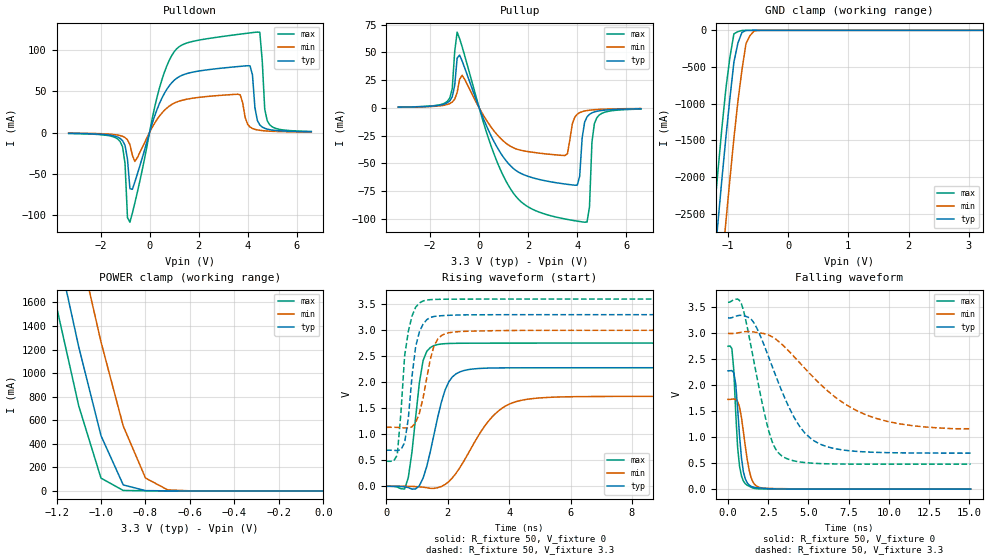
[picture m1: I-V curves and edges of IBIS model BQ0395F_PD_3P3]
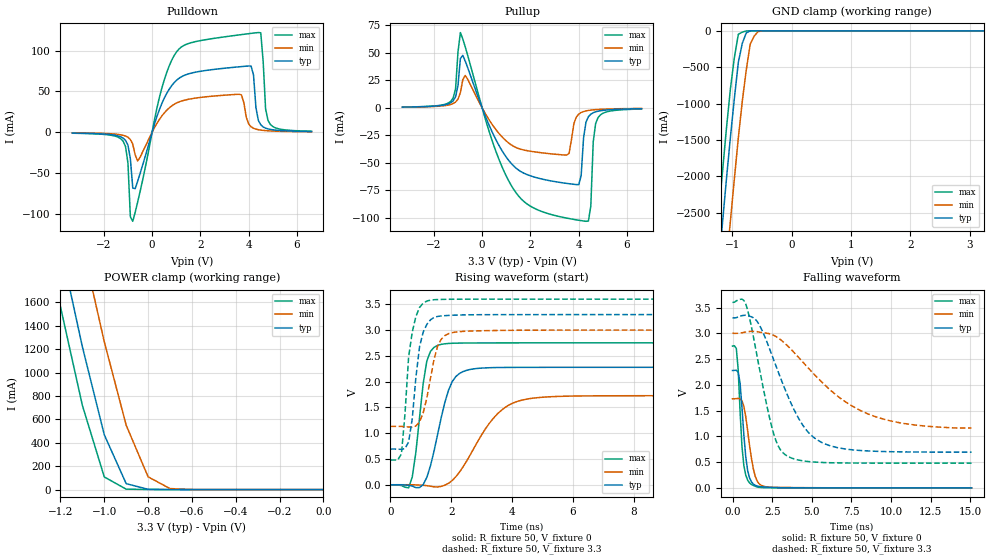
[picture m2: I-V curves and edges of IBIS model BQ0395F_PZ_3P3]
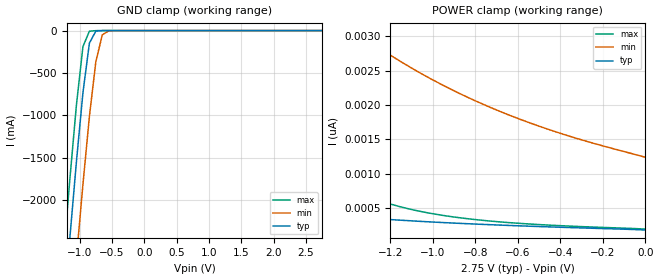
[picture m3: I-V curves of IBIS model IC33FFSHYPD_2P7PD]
[IBIS Ver]   3.2
[File Name]   sprm398.ibs
[File Rev]   1.0
[Date]   February 11, 2008
[Source]   File originated at Texas Instruments
[Copyright]   (c) 2008, Texas Instruments Inc.
[Component]   f2802xpt
[Manufacturer] Texas Instruments
[Package]
| Variable   Typ   Min   Max
R_pkg   0.277   0.133   0.378
L_pkg   1.76e-09   1.23e-09   2.19e-09
C_pkg   0.146e-12   0.05e-12   0.274e-12
[Pin] signal_name   model_name   R_pin   L_pin   C_pin
1   GPIO29   BQ0395F   0.284  1.74e-09  0.121e-12
2   TRSTn   IC33FFSHYPD   0.254  1.59e-09  0.167e-12
3   XRSn   BC3350BFODHYPU   0.134  1.23e-09  0.172e-12
4   ADCINA6   NC   0.290  1.69e-09  0.156e-12
5   ADCINA4   NC   0.150  1.46e-09  0.167e-12
6   ADCINA7   NC   0.260  1.67e-09  0.094e-12
7   ADCINA3   NC   0.248  1.54e-09  0.139e-12
8   ADCINA1   NC   0.244  1.53e-09  0.145e-12
9   ADCINA2   NC   0.252  1.51e-09  0.153e-12
10   ADCINA0   NC   0.151  1.39e-09  0.183e-12
11   VDDA   NC   0.286  1.83e-09  0.167e-12
12   VSSA   NC   0.163  1.61e-09  0.138e-12
13   ADCINB1   NC   0.315  1.87e-09  0.121e-12
14   ADCINB2   NC   0.314  1.84e-09  0.170e-12
15   ADCINB3   NC   0.317  1.870e-09 0.163e-12
16   ADCINB4   NC   0.323  1.86e-09  0.155e-12
17   ADCINB6   NC   0.330  1.80e-09  0.149e-12
18   ADCINB7   NC   0.343  1.86e-09  0.057e-12
19   GPIO34   BC3350AFHYPU   0.336  1.87e-09  0.085e-12
20   GPIO35   BC3350AFHYPU   0.335  1.88e-09  0.147e-12
21   GPIO36   BC3325CFHYPU   0.336  1.98e-09  0.156e-12
22   GPIO37   BC3325CFHYPU   0.338  2.03e-09  0.164e-12
23   GPIO38   BC3350AFHYPU   0.337  1.94e-09  0.171e-12
24   GPIO18   BQ0395F   0.345  2.08e-09  0.123e-12
25   GPIO19   BC3325CFHYPU   0.291  1.82e-09  0.120e-12
26   GPIO17   BQ0395F   0.244  1.55e-09  0.167e-12
27   GPIO16   BQ0395F   0.238  1.48e-09  0.156e-12
28   GPIO1   BQ0483F   0.235  1.36e-09  0.149e-12
29   GPIO0   BQ0393F   0.242  1.51e-09  0.145e-12
30   TEST   NC   0.249  1.55e-09  0.089e-12
31   GPIO32   BQ0393F   0.247  1.55e-09  0.081e-12
32   VDD   NC   0.251  1.62e-09  0.145e-12
33   VSS   NC   0.264  1.57e-09  0.155e-12
34   VREGENZn   NC   0.297  1.80e-09  0.165e-12
35   VDDIO   NC   0.156  1.52e-09  0.184e-12
36   GPIO33   BQ0393F   0.285  1.72e-09  0.119e-12
37   GPIO2   BQ0393F   0.314  1.95e-09  0.124e-12
38   GPIO3   BQ0393F   0.314  1.96e-09  0.175e-12
39   GPIO4   BQ0393F   0.324  1.89e-09  0.167e-12
40   GPIO5   BQ0393F   0.348  2.1e-09   0.159e-12
41   GPIO6   BQ0393F   0.346  2.09e-09  0.147e-12
42   GPIO7   BQ0393F   0.344  2.08e-09  0.085e-12
43   VDD   NC   0.133  1.64e-09  0.205e-12
44   VSS   NC   0.133  1.65e-09  0.207e-12
45   X1   NC   0.350  2.06e-09  0.163e-12
46   X2   NC   0.378  2.19e-09  0.171e-12
47   GPIO12   BQ0393F   0.315  1.95e-09  0.169e-12
48   GPIO28   BQ0395F   0.315  2.02e-09  0.1219e-12
| End of package information
[Component]   BQ0395F
[Manufacturer]   Texas Instruments
[Package]
|  variable   typ   min   max
R_pkg   0   0   0
L_pkg   0   0   0
C_pkg   0   0   0
[Pin]   signal_name   model_name   R_pin   L_pin   C_pin
VSS   VSS   GND
VDDS   VDDS   POWER
PAD   PAD   BQ0395F
[Model Selector] BQ0395F
BQ0395F_PD_3P3  Cell operated at 3.3(nom)
|BQ0395F_PD_3P3; PULLDOWN_ON
BQ0395F_PZ_3P3  Cell operated at 3.3(nom)
[Component]   IC33FFSHYPD
[Manufacturer]   Texas Instruments.
[Package]
| variable   typ   min   max
R_pkg   0.000   0.000   0.000
L_pkg   0.000H   0.000H   0.000H
C_pkg   0.000F   0.000F   0.000F
[Pin]  signal_name   model_name   R_pin   L_pin   C_pin
PAD   PAD   IC33FFSHYPD_3P3PD
| Y   Y   dummy
VSS   VSS   GND
VDDS   VDDS   POWER
[Model Selector]  IC33FFSHYPD
IC33FFSHYPD_2P7PD   cell with PI=0 and VDDS as 2.75(typ)
IC33FFSHYPD_2P7PDZ   cell with PI=1 and VDDS as 2.75(typ)
IC33FFSHYPD_3P3PD   cell with PI=0 and VDDS as 3.3(typ)
IC33FFSHYPD_3P3PDZ   cell with PI=1 and VDDS as 3.3(typ)
|   Component IC33FFSHYPU
[Component]   BC3350BFODHYPU
[Manufacturer]   Texas Instruments.
[Package]
| variable   typ   min   max
R_pkg   0.000   0.000   0.000
L_pkg   0.000H   0.000H   0.000H
C_pkg   0.000F   0.000F   0.000F
[Pin]  signal_name   model_name   R_pin   L_pin   C_pin
PAD   PAD   BC3350BFODHYPU_3P3PU
| A   A   dummy
| GZ   GZ   dummy
| Y   Y   dummy
VSSS   VSSS   GND
VDDS   VDDS   POWER
[Model Selector]   BC3350BFODHYPU
BC3350BFODHYPU_2P5PU   cell   VDDS=2.75(TYP)
BC3350BFODHYPU_2P5PZ   cell   VDDS=2.75(TYP)
BC3350BFODHYPU_3P3PU   cell   VDDS=3.3(TYP)
BC3350BFODHYPU_3P3PZ   cell   VDDS=3.3(TYP)
|   Component IC33FFSHY
[Component]   BC3350AFHYPU
[Manufacturer]   Texas Instruments.
[Package]
| variable   typ   min   max
R_pkg   0.000   0.000   0.000
L_pkg   0.000H   0.000H   0.000H
C_pkg   0.000F   0.000F   0.000F
[Pin]  signal_name   model_name   R_pin   L_pin   C_pin
PAD   PAD   BC3350AFHYPU_3P3PU
| A   A   dummy
| GZ   GZ   dummy
| Y   Y   dummy
VSSS   VSSS   GND
VDDS   VDDS   POWER
[Model Selector]  BC3350AFHYPU
BC3350AFHYPU_2P5PU   cell   VDDS=2.5V(typ)  PI=0
BC3350AFHYPU_2P5PUZ  cell   VDDS=2.5V(typ)  PI=1
BC3350AFHYPU_3P3PU   cell   VDDS=3.3V(typ)  PI=0
BC3350AFHYPU_3P3PUZ  cell   VDDS=3.3V(typ)  PI=1
|   Component OC3325CF
[Component]   BC3325CFHYPU
[Manufacturer]   Texas Instruments.
[Package]
| variable   typ   min   max
R_pkg   0.000   0.000   0.000
L_pkg   0.000H   0.000H   0.000H
C_pkg   0.000F   0.000F   0.000F
[Pin]  signal_name   model_name   R_pin   L_pin   C_pin
PAD   PAD   BC3325CFHYPU_3P3PU
| A   A   dummy
| GZ   GZ   dummy
| Y   Y   dummy
VSSS   VSSS   GND
VDDS   VDDS   POWER
[Model Selector]   BC3325CFHYPU
BC3325CFHYPU_2P5PU   cell  VDDS=2.75(TYP)  PI=0
BC3325CFHYPU_2P5PUZ   cell  VDDS=2.75(TYP)  PI=1
BC3325CFHYPU_3P3PU   cell  VDDS=3.3(TYP)  PI=0
BC3325CFHYPU_3P3PUZ   cell  VDDS=3.3(TYP)  PI=1
|   Component BC3350AFHYPU
[Component]   BQ0483F
[Manufacturer]   Texas Instruments
[Package]
|  variable   typ   min   max
R_pkg   0   0   0
L_pkg   0   0   0
C_pkg   0   0   0
[Pin]   signal_name   model_name   R_pin   L_pin   C_pin
VSS   VSS   GND
VDDS   VDDS   POWER
PAD   PAD   BQ0483F
[Model Selector] BQ0483F
BQ0483F_PD_3P3  Cell operated at 3.3(nom)
|BQ0483F_PD_3P3; PULLDOWN_ON
BQ0483F_PZ_3P3  Cell operated at 3.3(nom)
[Component]   BQ0393F
[Manufacturer]   Texas Instruments
[Package]
|  variable   typ   min   max
R_pkg   0   0   0
L_pkg   0   0   0
C_pkg   0   0   0
[Pin]   signal_name   model_name   R_pin   L_pin   C_pin
VSS   VSS   GND
VDDS   VDDS   POWER
PAD   PAD   BQ0393F
[Model Selector] BQ0393F
BQ0393F_PD_3P3  Cell operated at 3.3(nom)
|BQ0393F_PD_3P3; PULLDOWN_ON
BQ0393F_PZ_3P3  Cell operated at 3.3(nom)
| Models and submodels in the file (22): BQ0395F_PD_3P3 (I/O), BQ0395F_PZ_3P3 (I/O), IC33FFSHYPD_2P7PD (Input), IC33FFSHYPD_2P7PDZ (Input), IC33FFSHYPD_3P3PD (Input), IC33FFSHYPD_3P3PDZ (Input), BC3350BFODHYPU_2P5PU (I/O_open_drain), BC3350BFODHYPU_2P5PZ (I/O_open_drain), BC3350BFODHYPU_3P3PU (I/O_open_drain), BC3350BFODHYPU_3P3PZ (I/O_open_drain), BC3350AFHYPU_2P5PU (I/O), BC3350AFHYPU_2P5PUZ (I/O), BC3350AFHYPU_3P3PU (I/O), BC3350AFHYPU_3P3PUZ (I/O), BC3325CFHYPU_2P5PU (I/O), BC3325CFHYPU_2P5PUZ (I/O), BC3325CFHYPU_3P3PU (I/O), BC3325CFHYPU_3P3PUZ (I/O), BQ0483F_PD_3P3 (I/O), BQ0483F_PZ_3P3 (I/O), BQ0393F_PD_3P3 (I/O), BQ0393F_PZ_3P3 (I/O)
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|BQ0395F_PZ_3P3; PULLDOWN_OFF
|   Model Cell BQ0395F_PD_3P3
|BQ0395F_PD_3P3
[Model]   BQ0395F_PD_3P3
Model_type   I/O
Polarity   Non-Inverting
Enable   Active-Low
Vinl =  1.15
Vinh =  1.65
Cref =  15.0001pF
Rref =  101.0000M
Vref =  0V
Vmeas =  1.65
C_comp   1.2p   1.2p   1.2p
[Model Spec]
Vinl   1.15   1.05   1.15
Vinh   1.65   1.65   1.65
[Temperature Range]   25   125   -40
[Voltage Range]   3.3   3   3.6
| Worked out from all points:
|   slope of the pulldown table from 0 to 0.495 V, typ, clamps not added: 12 ohm
|   slope of the pullup table from 0 to 0.495 V, typ, clamps not added: 19.4 ohm
|   GND clamp passes 1 mA (typ) near -0.66 V on its own axis
|   POWER clamp passes 1 mA (typ) near -0.72 V on its own axis
|   rising waveform, R_fixture 50, V_fixture 0: 20-80 % time 553ps typ, 1.15ns min, 327ps max; typ from 0.001 V to 2.28 V
|   rising waveform, R_fixture 50, V_fixture 3.3: 20-80 % time 302ps typ, 400ps min, 286ps max; typ from 0.695 V to 3.3 V
|   falling waveform, R_fixture 50, V_fixture 0: 20-80 % time 372ps typ, 499ps min, 308ps max; typ from 2.28 V to 0.001 V
|   falling waveform, R_fixture 50, V_fixture 3.3: 20-80 % time 2.21ns typ, 4.03ns min, 1.26ns max; typ from 3.3 V to 0.695 V
[POWER_clamp]
|   voltage   I(typ)   I(min)   I(max)
-3.3V     22.47A     23.26A     22.03A
-1.233V   2.386A     3.273A     1.866A
-1.2V     2.084A     2.97A      1.564A
-1.167V   1.796A     2.677A     1.283A
-1.133V   1.509A     2.384A     1.002A
-1.067V   970.3mA    1.815A     516.3mA
-1.033V   719.4mA    1.539A     312.3mA
-1V       468.5mA    1.264A     108.3mA
-900mV    50.9mA     550mA      3.945mA
-800mV    2.599mA    109.2mA    1.152mA
-700mV    531.1uA    8.818mA    336.1uA
0V        279.6pA    1.919nA    325pA
[Pulldown]
|   voltage   I(typ)   I(min)   I(max)
-3.3V     -988.5uA   -708.3uA   -1.157mA
-1.2V     -7.098mA   -3.712mA   -10.91mA
-800mV    -68.22mA   -14.66mA   -108.9mA
-600mV    -60.07mA   -35.15mA   -85.64mA
300mV     27.57mA    15.61mA    42.26mA
1V        63.3mA     35.61mA    97.86mA
3.7V      80.34mA    45.74mA    119.5mA
4.1V      80.98mA    6.702mA    121mA
4.4V      14.6mA     3.158mA    122mA
4.5V      9.15mA     2.669mA    121.7mA
4.8V      4.146mA    1.814mA    14.51mA
6.6V      929.5uA    610.9uA    1.29mA
[Pullup]
|   voltage   I(typ)   I(min)   I(max)
-3.3V     680.2uA    582.8uA    724.9uA
-1.3V     4.616mA    3.102mA    5.939mA
-900mV    44.89mA    13.88mA    68.33mA
600mV     -30.17mA   -20.61mA   -41.26mA
1.7V      -59mA      -38.13mA   -84.39mA
3.5V      -68.55mA   -42.86mA   -100.1mA
4V        -69.63mA   -5.654mA   -102mA
4.3V      -12.95mA   -2.78mA    -103mA
4.5V      -5.735mA   -2.056mA   -89.2mA
4.6V      -4.432mA   -1.817mA   -30.89mA
4.8V      -3.028mA   -1.473mA   -8.825mA
6.6V      -767.6uA   -538uA     -1.05mA
[GND_clamp]
|   voltage   I(typ)   I(min)   I(max)
-3.3V     -23.4A     -24.5A     -22.76A
-1.3V     -3.866A    -5.045A    -3.159A
-1.233V   -3.247A    -4.425A    -2.54A
-1.167V   -2.635A    -3.811A    -1.931A
-1.033V   -1.46A     -2.609A    -794.5mA
-966.7mV  -926.2mA   -2.032A    -365.7mA
-900mV    -431.8mA   -1.469A    -47.48mA
-833.3mV  -172mA     -967.1mA   -17.77mA
-766.7mV  -28.5mA    -538.6mA   -2.104mA
-700mV    -1.454mA   -183.8mA   -472.2uA
-566.7mV  -175.9uA   -11.4mA    -230.7uA
3.233V    -8.123uA   19.88uA    -59.92uA
[Ramp]
| variable   typ   min   max
dV/dt_f   2.125235/3.393203n   1.522792/6.529444n   2.546199/1.871013n
dV/dt_r   1.870375/0.8633114n   1.417739/1.795571n   2.257927/0.4923715n
R_load = 50
[Rising Waveform]
R_fixture = 50
V_fixture = 0
V_fixture_min = 0
V_fixture_max = 0
|   time   V(typ)   V(min)   V(max)
0s        1.011mV    996.9uV    1.133mV
600ps     -10.22mV   1.405mV    -51.04mV
720ps     -23.4mV    678.7uV    169.5mV
1.2ns     155.9mV    -16.37mV   2.416V
1.556ns   996.6mV    -39.43mV   2.707V
1.916ns   1.849V     34.62mV    2.743V
2.276ns   2.164V     253.6mV    2.749V
3.44ns    2.275V     1.329V     2.753V
4.344ns   2.279V     1.646V     2.753V
15.09ns   2.28V      1.73V      2.754V
[Rising Waveform]
R_fixture = 50
V_fixture = 3.3
V_fixture_min = 3
V_fixture_max = 3.6
|   time   V(typ)   V(min)   V(max)
0s        694.6mV    1.135V     482.1mV
360ps     687.7mV    1.134V     601.7mV
480ps     707.3mV    1.129V     1.417V
600ps     840mV      1.123V     2.509V
720ps     1.306V     1.122V     2.977V
960ps     2.69V      1.227V     3.444V
1.2ns     3.117V     1.697V     3.564V
1.556ns   3.265V     2.698V     3.593V
2.036ns   3.288V     2.952V     3.598V
15.09ns   3.3V       3V         3.6V
[Falling Waveform]
R_fixture = 50
V_fixture = 0
V_fixture_min = 0
V_fixture_max = 0
|   time   V(typ)   V(min)   V(max)
0s        2.28V      1.73V      2.753V
240ps     2.285V     1.734V     2.71V
360ps     2.243V     1.738V     2.295V
480ps     2.031V     1.73V      1.476V
720ps     1.017V     1.582V     435.1mV
960ps     332.5mV    1.104V     155.7mV
1.2ns     120.6mV    564.9mV    75.69mV
1.556ns   42.01mV    135.6mV    22.21mV
2.156ns   20.25mV    22.83mV    5.408mV
15.09ns   1.097mV    1.119mV    1.182mV
[Falling Waveform]
R_fixture = 50
V_fixture = 3.3
V_fixture_min = 3
V_fixture_max = 3.6
|   time   V(typ)   V(min)   V(max)
0s        3.3V       3V         3.599V
840ps     3.35V      3.025V     3.566V
1.556ns   3.23V      3.032V     2.552V
2.516ns   2.556V     2.972V     1.143V
2.876ns   2.261V     2.911V     824.8mV
3.328ns   1.906V     2.798V     645.9mV
4.792ns   1.077V     2.324V     512.9mV
6.208ns   814.6mV    1.891V     489.5mV
9.672ns   706.3mV    1.325V     482.1mV
15.09ns   695.1mV    1.165V     482mV
|   Model Cell BQ0395F_PZ_3P3
|BQ0395F_PZ_3P3
[Model]   BQ0395F_PZ_3P3
Model_type   I/O
Polarity   Non-Inverting
Enable   Active-Low
Vinl =  1.15
Vinh =  1.65
Cref =  15.0001pF
Rref =  101.0000M
Vref =  0V
Vmeas =  1.65
C_comp   1.2p   1.2p   1.2p
[Model Spec]
Vinl   1.15   1.05   1.15
Vinh   1.65   1.65   1.65
[Temperature Range]   25   125   -40
[Voltage Range]   3.3   3   3.6
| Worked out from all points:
|   slope of the pulldown table from 0 to 0.495 V, typ, clamps not added: 12 ohm
|   slope of the pullup table from 0 to 0.495 V, typ, clamps not added: 19.3 ohm
|   GND clamp passes 1 mA (typ) near -0.68 V on its own axis
|   POWER clamp passes 1 mA (typ) near -0.73 V on its own axis
|   rising waveform, R_fixture 50, V_fixture 0: 20-80 % time 552ps typ, 1.15ns min, 326ps max; typ from 0 V to 2.28 V
|   rising waveform, R_fixture 50, V_fixture 3.3: 20-80 % time 301ps typ, 401ps min, 286ps max; typ from 0.693 V to 3.3 V
|   falling waveform, R_fixture 50, V_fixture 0: 20-80 % time 370ps typ, 499ps min, 306ps max; typ from 2.28 V to 0 V
|   falling waveform, R_fixture 50, V_fixture 3.3: 20-80 % time 2.2ns typ, 4.03ns min, 1.26ns max; typ from 3.3 V to 0.693 V
[POWER_clamp]
|   voltage   I(typ)   I(min)   I(max)
-3.3V     22.47A     23.26A     22.03A
-1.233V   2.386A     3.273A     1.866A
-1.2V     2.084A     2.97A      1.564A
-1.167V   1.796A     2.677A     1.283A
-1.133V   1.509A     2.384A     1.001A
-1.067V   970.3mA    1.815A     516.3mA
-1.033V   719.4mA    1.539A     312.3mA
-1V       468.5mA    1.264A     108.3mA
-900mV    50.85mA    550mA      3.793mA
-800mV    2.505mA    109.2mA    1.004mA
-700mV    437.8uA    8.783mA    205.6uA
0V        281.4pA    1.921nA    326.9pA
[Pulldown]
|   voltage   I(typ)   I(min)   I(max)
-3.3V     -988.5uA   -708.3uA   -1.157mA
-1.2V     -7.098mA   -3.712mA   -10.91mA
-800mV    -68.21mA   -14.66mA   -108.9mA
-600mV    -60.07mA   -35.15mA   -85.65mA
300mV     27.57mA    15.61mA    42.26mA
1V        63.3mA     35.61mA    97.86mA
3.7V      80.34mA    45.73mA    119.5mA
4.1V      80.98mA    6.702mA    121mA
4.4V      14.6mA     3.158mA    122mA
4.5V      9.15mA     2.669mA    121.7mA
4.8V      4.146mA    1.814mA    14.51mA
6.6V      929.5uA    610.9uA    1.29mA
[Pullup]
|   voltage   I(typ)   I(min)   I(max)
-3.3V     680.2uA    582.8uA    724.9uA
-1.3V     4.616mA    3.102mA    5.939mA
-900mV    44.88mA    13.88mA    68.33mA
600mV     -30.17mA   -20.61mA   -41.26mA
1.7V      -59mA      -38.13mA   -84.39mA
3.5V      -68.55mA   -42.86mA   -100.1mA
4V        -69.63mA   -5.654mA   -102mA
4.3V      -12.95mA   -2.78mA    -103mA
4.5V      -5.735mA   -2.056mA   -89.18mA
4.6V      -4.432mA   -1.817mA   -30.89mA
4.8V      -3.028mA   -1.473mA   -8.824mA
6.6V      -767.6uA   -538uA     -1.05mA
[GND_clamp]
|   voltage   I(typ)   I(min)   I(max)
-3.3V     -23.4A     -24.5A     -22.76A
-1.3V     -3.866A    -5.045A    -3.159A
-1.233V   -3.247A    -4.425A    -2.54A
-1.167V   -2.635A    -3.811A    -1.931A
-1.033V   -1.46A     -2.609A    -794.5mA
-966.7mV  -926.2mA   -2.032A    -365.6mA
-900mV    -431.8mA   -1.469A    -47.3mA
-833.3mV  -171.9mA   -967mA     -17.57mA
-766.7mV  -28.37mA   -538.6mA   -1.884mA
-700mV    -1.315mA   -183.8mA   -250.9uA
-566.7mV  -34.93uA   -11.32mA   -9.563uA
3.233V    268.2pA    281.8nA    247.8pA
[Ramp]
| variable   typ   min   max
dV/dt_f   2.127044/3.389099n   1.52501/6.522896n   2.547898/1.869267n
dV/dt_r   1.87233/0.8643675n   1.418387/1.796408n   2.260849/0.4926587n
R_load = 50
[Rising Waveform]
R_fixture = 50
V_fixture = 0
V_fixture_min = 0
V_fixture_max = 0
|   time   V(typ)   V(min)   V(max)
0s        -85.83uV   -72.94uV   -48.69uV
596ps     -11.15mV   351.6uV    -60.03mV
836ps     -56.28mV   -2.353mV   634.8mV
1.196ns   143.6mV    -17.49mV   2.401V
1.552ns   979.8mV    -43.14mV   2.703V
1.912ns   1.837V     29.22mV    2.741V
2.272ns   2.159V     246.3mV    2.747V
3.428ns   2.272V     1.317V     2.751V
4.328ns   2.277V     1.641V     2.752V
15.08ns   2.278V     1.727V     2.752V
[Rising Waveform]
R_fixture = 50
V_fixture = 3.3
V_fixture_min = 3
V_fixture_max = 3.6
|   time   V(typ)   V(min)   V(max)
0s        692.6mV    1.132V     480.3mV
360ps     685.7mV    1.131V     599.1mV
476ps     702.9mV    1.126V     1.367V
596ps     828.8mV    1.12V      2.476V
716ps     1.28V      1.119V     2.961V
956ps     2.675V     1.22V      3.439V
1.196ns   3.11V      1.681V     3.563V
1.552ns   3.265V     2.687V     3.592V
2.152ns   3.29V      2.962V     3.598V
15.08ns   3.3V       3V         3.6V
[Falling Waveform]
R_fixture = 50
V_fixture = 0
V_fixture_min = 0
V_fixture_max = 0
|   time   V(typ)   V(min)   V(max)
0s        2.278V     1.727V     2.751V
240ps     2.283V     1.732V     2.708V
360ps     2.241V     1.736V     2.291V
476ps     2.039V     1.728V     1.496V
716ps     1.028V     1.585V     434mV
956ps     333.3mV    1.11V      148.2mV
1.196ns   115.7mV    569.8mV    65.9mV
1.552ns   35.55mV    133.4mV    16.89mV
2.152ns   14.57mV    18.82mV    3.451mV
15.08ns   1.284uV    41.76uV    650.7nV
[Falling Waveform]
R_fixture = 50
V_fixture = 3.3
V_fixture_min = 3
V_fixture_max = 3.6
|   time   V(typ)   V(min)   V(max)
0s        3.3V       3V         3.599V
836ps     3.35V      3.024V     3.569V
1.552ns   3.232V     3.032V     2.555V
2.508ns   2.56V      2.973V     1.146V
2.98ns    2.174V     2.888V     758.9mV
3.428ns   1.828V     2.769V     622.7mV
4.776ns   1.079V     2.328V     511.4mV
6.192ns   813.2mV    1.893V     487.6mV
9.664ns   704.1mV    1.323V     480.2mV
15.08ns   693mV      1.162V     480.1mV
|   Model IC33FFSHYPD_2P7PD
[Model]   IC33FFSHYPD_2P7PD
Model_type   Input
Polarity   Non-Inverting
Vinl =   0.8250V
Vinh =   1.9250V
C_comp   2.1397pF   2.1767pF   2.7158pF
[Temperature Range]   25.0000   0.1250k   -40.0000
[Voltage Range]   2.7500V   2.5000V   3.0000V
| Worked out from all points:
|   GND clamp passes 1 mA (typ) near -0.66 V on its own axis
[GND_clamp]
| voltage   I(typ)   I(min)   I(max)
-2.75V    -17.91A    -19.01A    -17.27A
-1.25V    -3.342A    -4.502A    -2.646A
-1.15V    -2.424A    -3.58A     -1.732A
-1.05V    -1.541A    -2.68A     -871.7mA
-950mV    -732.7mA   -1.814A    -188.7mA
-850mV    -147.9mA   -1.014A    -7.752mA
-750mV    -6.009mA   -364.9mA   -798.7uA
-650mV    -206.4uA   -49.97mA   -59.18uA
-550mV    -9.486uA   -3.233mA   -2.615uA
2.75V     181.8pA    1.449nA    170.8pA
[POWER_clamp]
| voltage   I(typ)   I(min)   I(max)
-2.75V    1.398nA    9.161nA    24.63nA
-2.4V     922.6pA    6.884nA    9.415nA
-2V       612.2pA    5.001nA    3.237nA
-1.95V    584.8pA    4.808nA    2.846nA
-1.8V     512.9pA    4.278nA    1.955nA
-1.7V     472.6pA    3.961nA    1.538nA
-1.55V    421.6pA    3.534nA    1.095nA
-1.35V    367.1pA    3.045nA    729.7pA
-1.1V     315.3pA    2.541nA    480.7pA
-750mV    261.9pA    1.994nA    318pA
-400mV    222pA      1.589nA    244.9pA
0V        181.8pA    1.241nA    195.1pA
